(* Logix 5000 AddOnInstructionDefinition export POINT_DBL; software revision 30.00 *)

TYPE POINT :   // A point on an Edwards-curve represented in extended homogeneous coordinates
STRUCT
   X : DINT[22];
   Y : DINT[22];
   Z : DINT[22];
   T : DINT[22];
END_STRUCT
END_TYPE

ADD_ON_INSTRUCTION B256_ADD   (* revision 1.0 20170916, vendor Kenneth A. Fischer *)
// c3=c1+c2 with no reduction
// Revision note:
// Rev1.0: 20170916 - Initial Release
VAR_IN_OUT
   Inp_C1 : DINT[22]; {required}
   Inp_C2 : DINT[22]; {required}
   Out_C3 : DINT[22]; {required}
END_VAR
VAR
   i : INT;
END_VAR

ROUTINE Logic   (* ladder *)
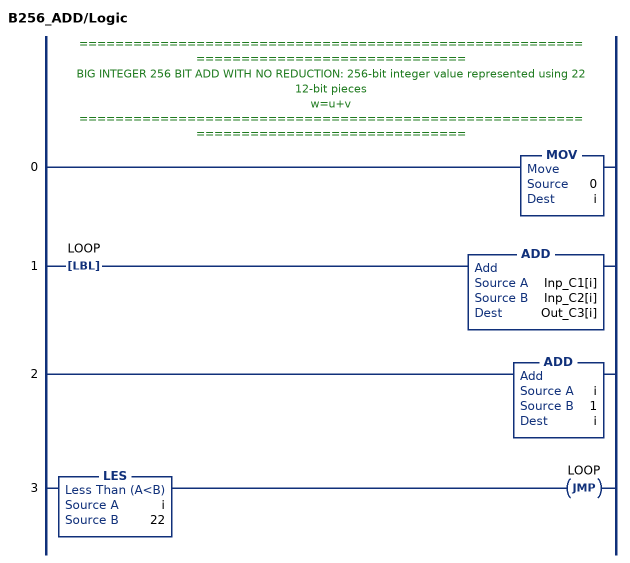
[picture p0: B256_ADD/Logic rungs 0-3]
   // ======================================================================================
   // BIG INTEGER 256 BIT ADD WITH NO REDUCTION: 256-bit integer value represented using 22 12-bit pieces
   // w=u+v
   // ======================================================================================
   0: MOV(0,i);
   1: LBL(LOOP)ADD(Inp_C1[i],Inp_C2[i],Out_C3[i]);
   2: ADD(i,1,i);
   3: LES(i,22)JMP(LOOP);
END_ROUTINE
END_ADD_ON_INSTRUCTION

ADD_ON_INSTRUCTION D_SHR   (* revision 1.0 20170524, vendor Kenneth A. Fischer *)
// DINT bit shift right of the 32-bit argument Inp_A by Inp_B bits with paddding by zeros on the right
// Revision note:
// Rev1.0: 20170524 - Initial Release
VAR_IN_OUT
   Inp_A : DINT; {required}   // 64-bit Integer to be right circular rotated
END_VAR
VAR_INPUT
   Inp_B : INT; {required}   // Number of bits to shift
END_VAR
VAR_IN_OUT
   Out : DINT; {required}   // Result
END_VAR
VAR
   BSR_Cntrl : CONTROL := (LEN := 32);
   ONS : BOOL;
   Source_Bit : BOOL;
   Wrk_InpA : DINT[2];
END_VAR

ROUTINE Logic   (* ladder *)
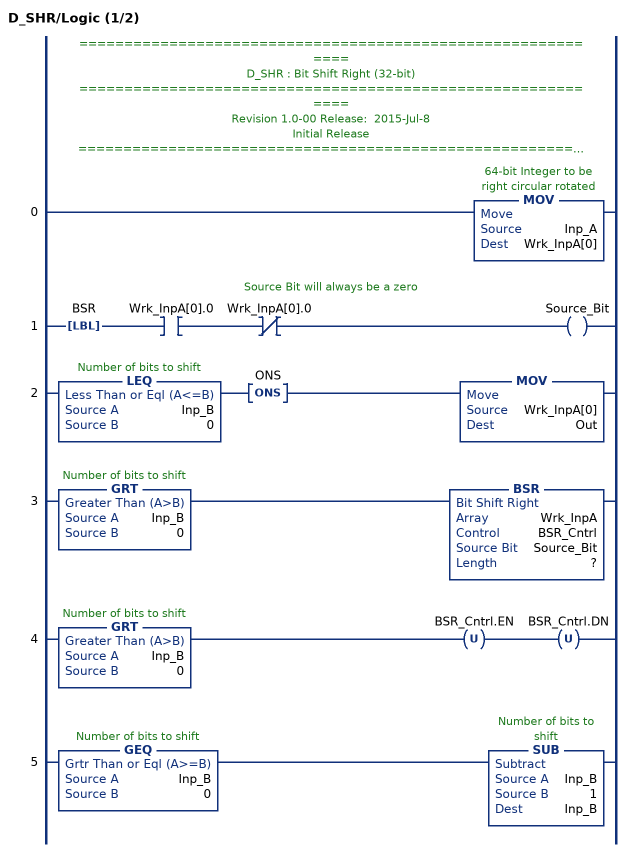
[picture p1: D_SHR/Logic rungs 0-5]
   // ============================================================
   // D_SHR : Bit Shift Right (32-bit)
   // ============================================================
   // Revision 1.0-00 Release:  2015-Jul-8
   // Initial Release
   // ============================================================
   // Performs a right bit shift of the 32-bit argument Inp_A by the
   // number of bits defined in the 16-bit argument Inp_B, with padding by zeros.
   0: MOV(Inp_A,Wrk_InpA[0]);
   // Source Bit will always be a zero
   1: LBL(BSR)XIC(Wrk_InpA[0].0)XIO(Wrk_InpA[0].0)OTE(Source_Bit);
   2: LEQ(Inp_B,0)ONS(ONS)MOV(Wrk_InpA[0],Out);
   3: GRT(Inp_B,0)BSR(Wrk_InpA,BSR_Cntrl,Source_Bit,?);
   4: GRT(Inp_B,0)OTU(BSR_Cntrl.EN)OTU(BSR_Cntrl.DN);
   5: GEQ(Inp_B,0)SUB(Inp_B,1,Inp_B);
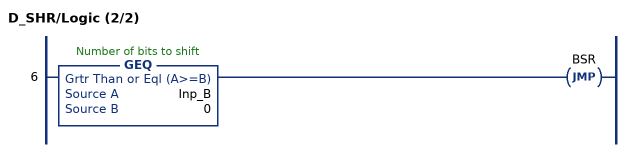
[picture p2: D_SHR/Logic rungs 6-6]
   6: GEQ(Inp_B,0)JMP(BSR);
END_ROUTINE
END_ADD_ON_INSTRUCTION

ADD_ON_INSTRUCTION B256_NRED   (* revision 1.0 20170916, vendor Kenneth A. Fischer *)
// Reduce 256-bit integer stored in 22 pieces by propagating carries
// Revision note:
// Rev1.0: 20170916 - Initial Release
VAR_IN_OUT
   Inp_C : DINT[22]; {required}
END_VAR
VAR
   D_SHR : D_SHR;
   temp : DINT;
   i : INT;
END_VAR

ROUTINE Logic   (* ladder *)
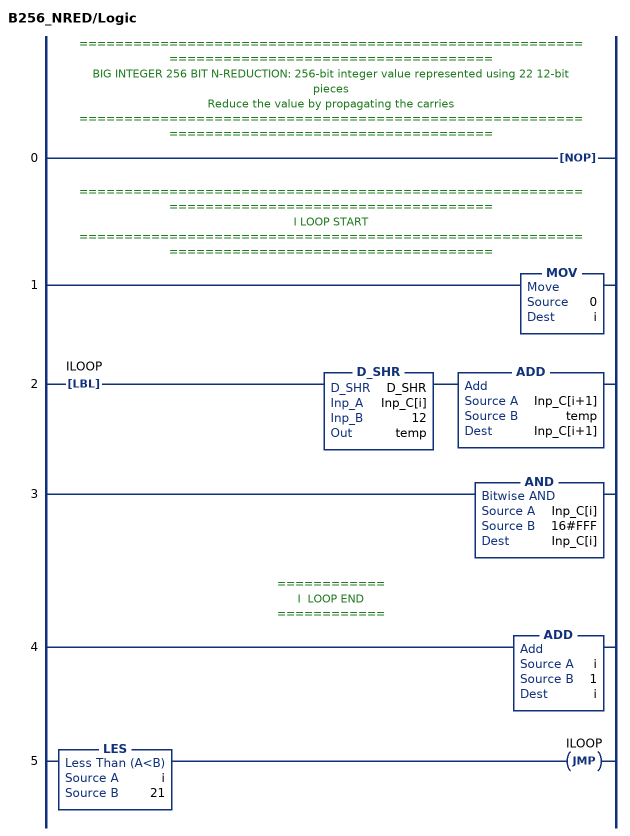
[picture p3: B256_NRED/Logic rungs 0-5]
   // ============================================================================================
   // BIG INTEGER 256 BIT N-REDUCTION: 256-bit integer value represented using 22 12-bit pieces
   // Reduce the value by propagating the carries
   // ============================================================================================
   0: NOP();
   // ============================================================================================
   // I LOOP START
   // ============================================================================================
   1: MOV(0,i);
   2: LBL(ILOOP)D_SHR(D_SHR,Inp_C[i],12,temp)ADD(Inp_C[i+1],temp,Inp_C[i+1]);
   3: AND(Inp_C[i],16#FFF,Inp_C[i]);
   // ============
   // I  LOOP END
   // ============
   4: ADD(i,1,i);
   5: LES(i,21)JMP(ILOOP);
END_ROUTINE
END_ADD_ON_INSTRUCTION

ADD_ON_INSTRUCTION B256_SUB   (* revision 1.0 20170916, vendor Kenneth A. Fischer *)
// c3=c1-c2 with reduction
// Revision note:
// Rev1.0: 20170916 - Initial Release
VAR_IN_OUT
   Inp_C1 : DINT[22]; {required}
   Inp_C2 : DINT[22]; {required}
   Out_C3 : DINT[22]; {required}
END_VAR
VAR
   B256_ADD : B256_ADD;
   B256_NRED : B256_NRED;
   temp : DINT;
   i : INT;
END_VAR

ROUTINE Logic   (* ladder *)
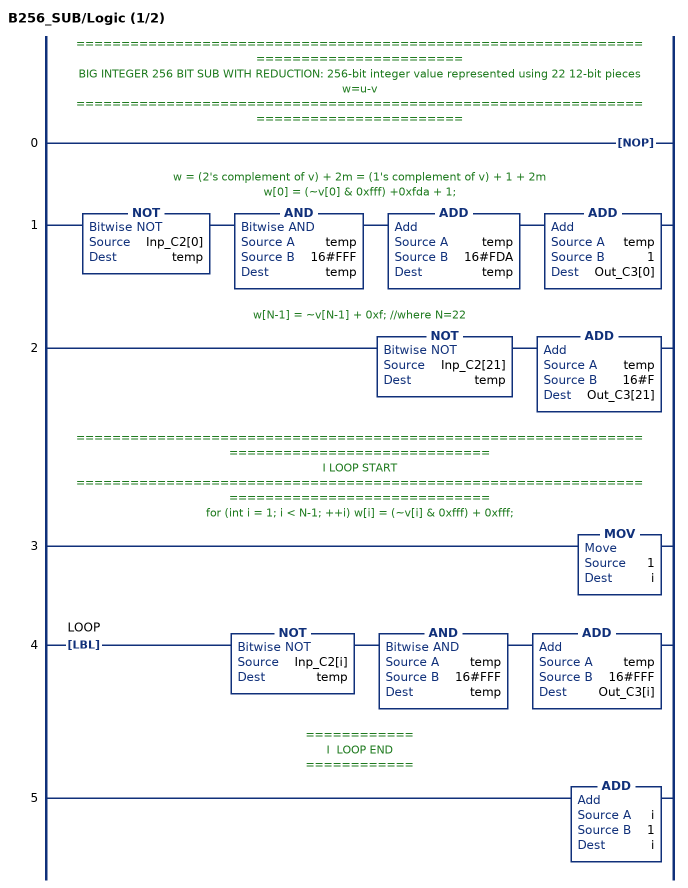
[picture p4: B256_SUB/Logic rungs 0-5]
   // ======================================================================================
   // BIG INTEGER 256 BIT SUB WITH REDUCTION: 256-bit integer value represented using 22 12-bit pieces
   //  w=u-v
   // ======================================================================================
   0: NOP();
   // w = (2's complement of v) + 2m = (1's complement of v) + 1 + 2m
   // w[0] = (~v[0] & 0xfff) +0xfda + 1;
   1: NOT(Inp_C2[0],temp)AND(temp,16#FFF,temp)ADD(temp,16#FDA,temp)ADD(temp,1,Out_C3[0]);
   // w[N-1] = ~v[N-1] + 0xf; //where N=22
   2: NOT(Inp_C2[21],temp)ADD(temp,16#F,Out_C3[21]);
   // ============================================================================================
   // I LOOP START
   // ============================================================================================
   // for (int i = 1; i < N-1; ++i) w[i] = (~v[i] & 0xfff) + 0xfff;
   3: MOV(1,i);
   4: LBL(LOOP)NOT(Inp_C2[i],temp)AND(temp,16#FFF,temp)ADD(temp,16#FFF,Out_C3[i]);
   // ============
   // I  LOOP END
   // ============
   5: ADD(i,1,i);
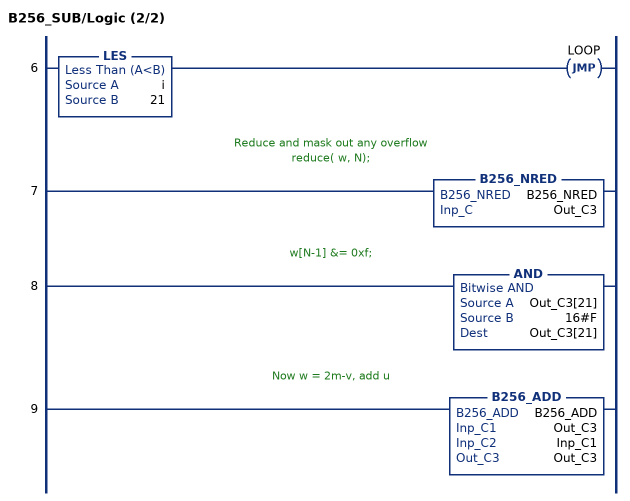
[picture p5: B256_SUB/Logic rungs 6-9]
   6: LES(i,21)JMP(LOOP);
   // Reduce and mask out any overflow
   // reduce( w, N);
   7: B256_NRED(B256_NRED,Out_C3);
   // w[N-1] &= 0xf;
   8: AND(Out_C3[21],16#F,Out_C3[21]);
   // Now w = 2m-v, add u
   9: B256_ADD(B256_ADD,Out_C3,Inp_C1,Out_C3);
END_ROUTINE
END_ADD_ON_INSTRUCTION

ADD_ON_INSTRUCTION B256_FRED   (* revision 1.0 20170916, vendor Kenneth A. Fischer *)
// fast_reduce:  reduce by propagating the carries starting at a particular offset and stoping once the carry becomes zero
// Revision note:
// Rev1.0: 20170916 - Initial Release
VAR_IN_OUT
   Inp_C : DINT[22]; {required}
END_VAR
VAR_INPUT
   Inp_offset : INT; {required}
END_VAR
VAR
   i : INT;
   carry : DINT;
   D_SHR : D_SHR;
END_VAR

ROUTINE Logic   (* ladder *)
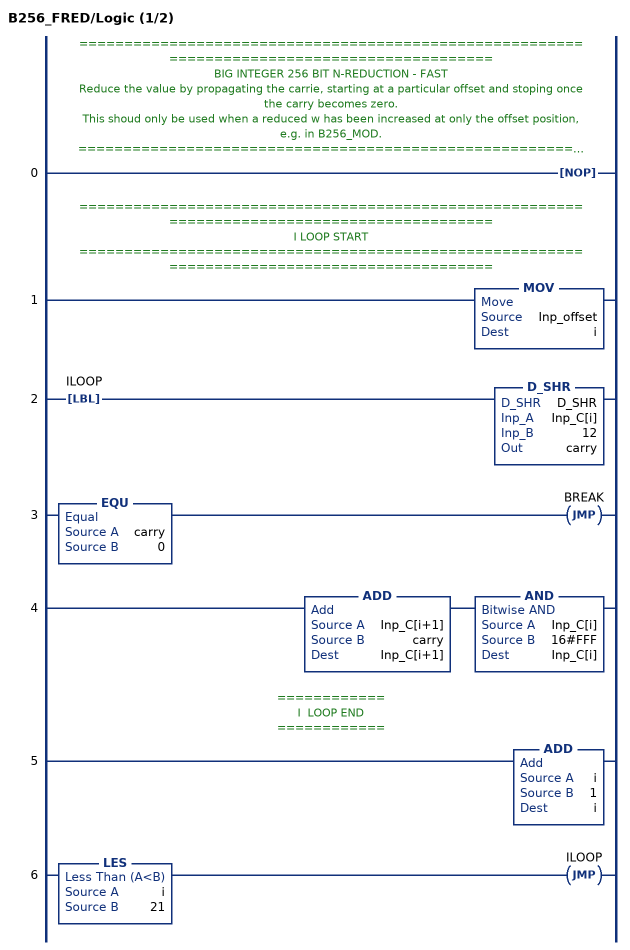
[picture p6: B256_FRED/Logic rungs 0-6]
   // ============================================================================================
   // BIG INTEGER 256 BIT N-REDUCTION - FAST
   // Reduce the value by propagating the carrie, starting at a particular offset and stoping once the carry becomes zero.
   // This shoud only be used when a reduced w has been increased at only the offset position, e.g. in B256_MOD.
   // ============================================================================================
   0: NOP();
   // ============================================================================================
   // I LOOP START
   // ============================================================================================
   1: MOV(Inp_offset,i);
   2: LBL(ILOOP)D_SHR(D_SHR,Inp_C[i],12,carry);
   3: EQU(carry,0)JMP(BREAK);
   4: ADD(Inp_C[i+1],carry,Inp_C[i+1])AND(Inp_C[i],16#FFF,Inp_C[i]);
   // ============
   // I  LOOP END
   // ============
   5: ADD(i,1,i);
   6: LES(i,21)JMP(ILOOP);
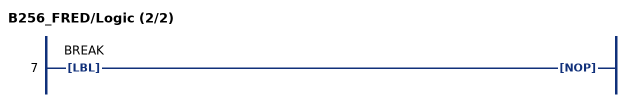
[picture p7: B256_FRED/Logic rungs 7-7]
   7: LBL(BREAK)NOP();
END_ROUTINE
END_ADD_ON_INSTRUCTION

ADD_ON_INSTRUCTION D_SHL   (* revision 1.0 20170524, vendor Kenneth A. Fischer *)
// DINT bit shift left of the 32-bit argument Inp_A by Inp_B bits with paddding by zeros on the right
// Revision note:
// Rev1.0: 20170524 - Initial Release
VAR_IN_OUT
   Inp_A : DINT; {required}   // 64-bit Integer to be right circular rotated
END_VAR
VAR_INPUT
   Inp_B : INT; {required}   // Number of bits to shift
END_VAR
VAR_IN_OUT
   Out : DINT; {required}   // Result
END_VAR
VAR
   Wrk_InpA : DINT[2];
   Source_Bit : BOOL;
   ONS : BOOL;
   BSL_Cntrl : CONTROL := (LEN := 32);
END_VAR

ROUTINE Logic   (* ladder *)
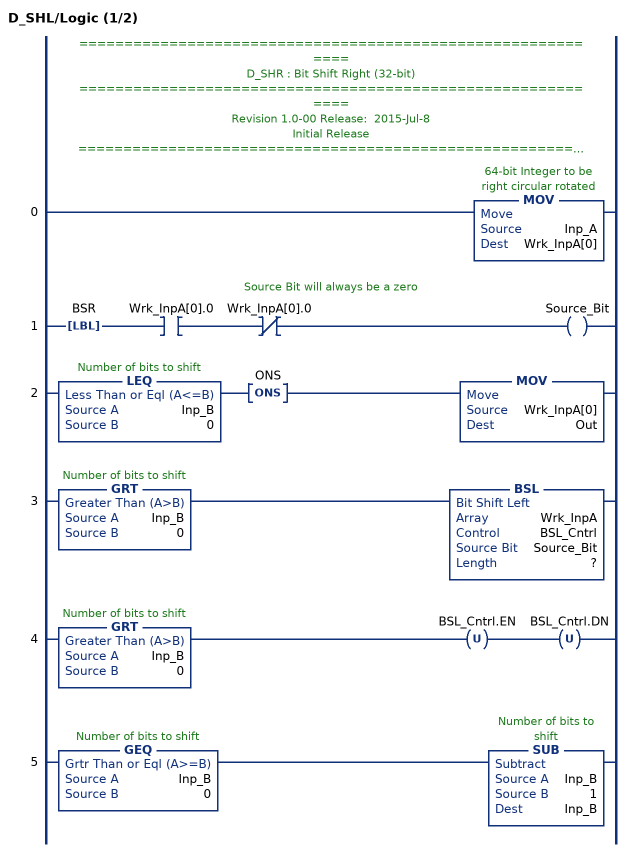
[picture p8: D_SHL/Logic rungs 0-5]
   // ============================================================
   // D_SHR : Bit Shift Right (32-bit)
   // ============================================================
   // Revision 1.0-00 Release:  2015-Jul-8
   // Initial Release
   // ============================================================
   // Performs a left bit shift of the 32-bit argument Inp_A by the
   // number of bits defined in the 16-bit argument Inp_B, with padding by zeros.
   0: MOV(Inp_A,Wrk_InpA[0]);
   // Source Bit will always be a zero
   1: LBL(BSR)XIC(Wrk_InpA[0].0)XIO(Wrk_InpA[0].0)OTE(Source_Bit);
   2: LEQ(Inp_B,0)ONS(ONS)MOV(Wrk_InpA[0],Out);
   3: GRT(Inp_B,0)BSL(Wrk_InpA,BSL_Cntrl,Source_Bit,?);
   4: GRT(Inp_B,0)OTU(BSL_Cntrl.EN)OTU(BSL_Cntrl.DN);
   5: GEQ(Inp_B,0)SUB(Inp_B,1,Inp_B);
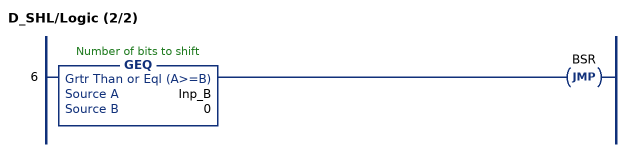
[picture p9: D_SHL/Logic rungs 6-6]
   6: GEQ(Inp_B,0)JMP(BSR);
END_ROUTINE
END_ADD_ON_INSTRUCTION

ADD_ON_INSTRUCTION B256_MOD   (* revision 1.0 20170916, vendor Kenneth A. Fischer *)
// c = d mod (2^255 - 19)
// Revision note:
// Rev1.0: 20170916 - Initial Release
VAR_IN_OUT
   Inp_D : DINT[43]; {required}
   Out_C : DINT[22]; {required}
END_VAR
VAR
   B256_NRED : B256_NRED;
   D_SHL : D_SHL;
   D_SHR : D_SHR;
   i : INT;
   t : DINT;
   temp : DINT;
   temp2 : DINT;
   B256_FRED : B256_FRED;
   offset : DINT;
END_VAR

ROUTINE Logic   (* ladder *)
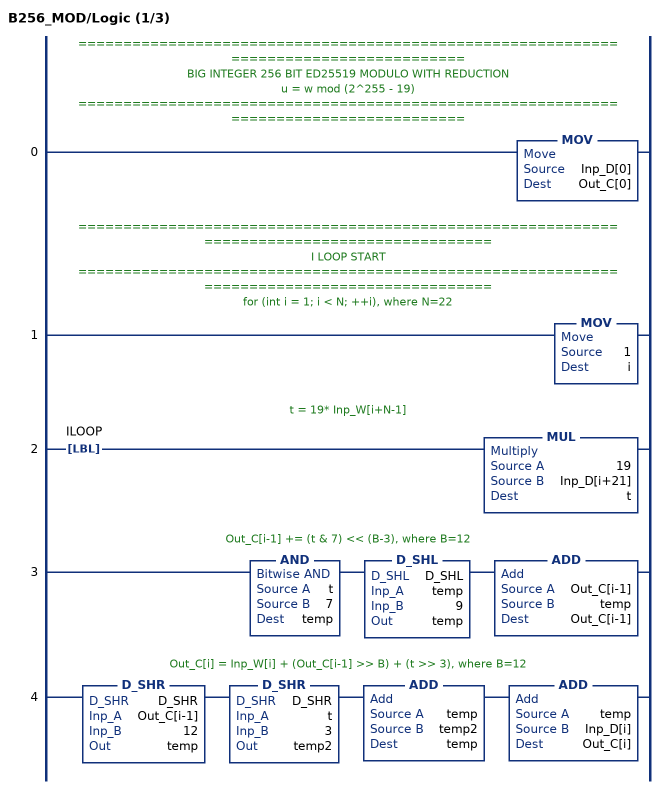
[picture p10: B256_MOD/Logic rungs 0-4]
   // ======================================================================================
   // BIG INTEGER 256 BIT ED25519 MODULO WITH REDUCTION
   //  u = w mod (2^255 - 19)
   // ======================================================================================
   0: MOV(Inp_D[0],Out_C[0]);
   // ============================================================================================
   // I LOOP START
   // ============================================================================================
   // for (int i = 1; i < N; ++i), where N=22
   1: MOV(1,i);
   // t = 19* Inp_W[i+N-1]
   2: LBL(ILOOP)MUL(19,Inp_D[i+21],t);
   // Out_C[i-1] += (t & 7) << (B-3), where B=12
   3: AND(t,7,temp)D_SHL(D_SHL,temp,9,temp)ADD(Out_C[i-1],temp,Out_C[i-1]);
   // Out_C[i] = Inp_W[i] + (Out_C[i-1] >> B) + (t >> 3), where B=12
   4: D_SHR(D_SHR,Out_C[i-1],12,temp)D_SHR(D_SHR,t,3,temp2)ADD(temp,temp2,temp)ADD(temp,Inp_D[i],Out_C[i]);
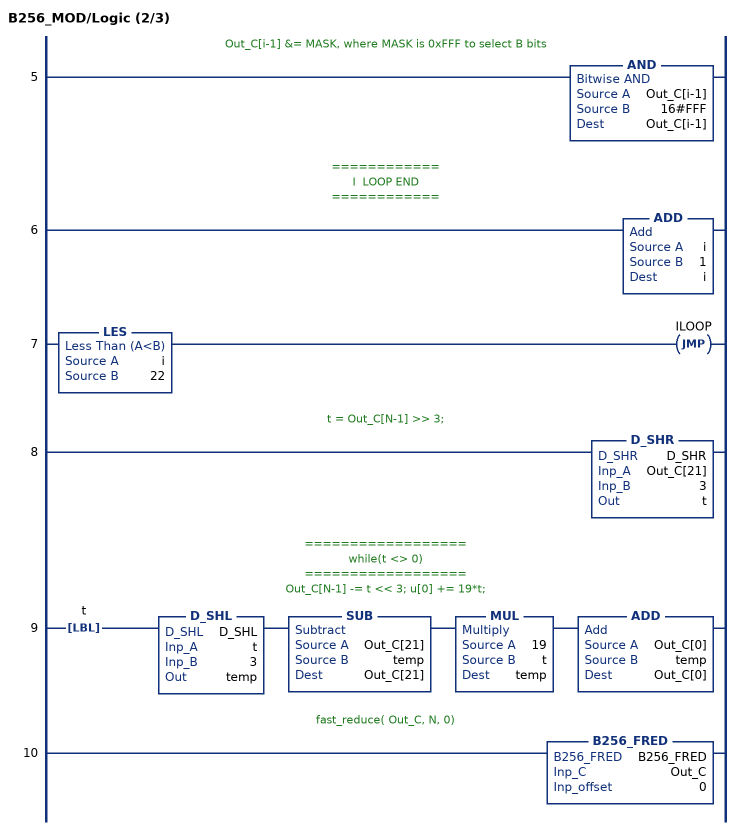
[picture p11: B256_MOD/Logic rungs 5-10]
   // Out_C[i-1] &= MASK, where MASK is 0xFFF to select B bits
   5: AND(Out_C[i-1],16#FFF,Out_C[i-1]);
   // ============
   // I  LOOP END
   // ============
   6: ADD(i,1,i);
   7: LES(i,22)JMP(ILOOP);
   // t = Out_C[N-1] >> 3;
   8: D_SHR(D_SHR,Out_C[21],3,t);
   // ==================
   // while(t <> 0)
   // ==================
   // Out_C[N-1] -= t << 3; u[0] += 19*t;
   9: LBL(t)D_SHL(D_SHL,t,3,temp)SUB(Out_C[21],temp,Out_C[21])MUL(19,t,temp)ADD(Out_C[0],temp,Out_C[0]);
   // fast_reduce( Out_C, N, 0)
   10: B256_FRED(B256_FRED,Out_C,0);
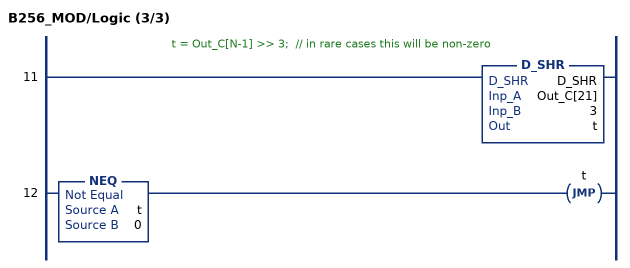
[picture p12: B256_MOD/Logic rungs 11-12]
   // t = Out_C[N-1] >> 3;  // in rare cases this will be non-zero
   11: D_SHR(D_SHR,Out_C[21],3,t);
   12: NEQ(t,0)JMP(t);
END_ROUTINE
END_ADD_ON_INSTRUCTION

ADD_ON_INSTRUCTION B256_NNRED   (* revision 1.0 20170916, vendor Kenneth A. Fischer *)
// Reduce 256-bit integer stored in 43 pieces by propagating carries
// Revision note:
// Rev1.0: 20170916 - Initial Release
VAR_IN_OUT
   Inp_D : DINT[43]; {required}
END_VAR
VAR
   temp : DINT;
   i : INT;
   D_SHR : D_SHR;
END_VAR

ROUTINE Logic   (* ladder *)
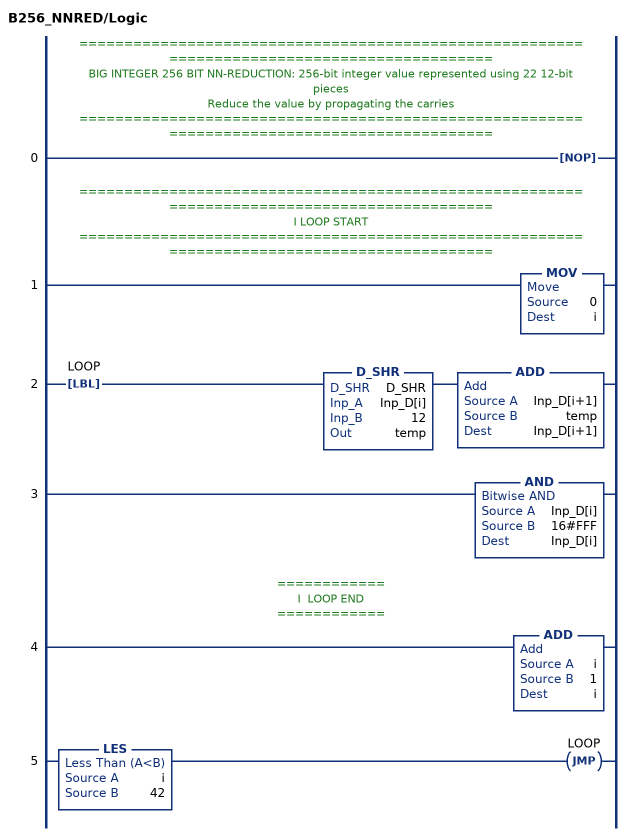
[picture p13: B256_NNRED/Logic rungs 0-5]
   // ============================================================================================
   // BIG INTEGER 256 BIT NN-REDUCTION: 256-bit integer value represented using 22 12-bit pieces
   // Reduce the value by propagating the carries
   // ============================================================================================
   0: NOP();
   // ============================================================================================
   // I LOOP START
   // ============================================================================================
   1: MOV(0,i);
   2: LBL(LOOP)D_SHR(D_SHR,Inp_D[i],12,temp)ADD(Inp_D[i+1],temp,Inp_D[i+1]);
   3: AND(Inp_D[i],16#FFF,Inp_D[i]);
   // ============
   // I  LOOP END
   // ============
   4: ADD(i,1,i);
   5: LES(i,42)JMP(LOOP);
END_ROUTINE
END_ADD_ON_INSTRUCTION

ADD_ON_INSTRUCTION B256_MUL   (* revision 1.0 20170916, vendor Kenneth A. Fischer *)
// c3 = c1*c2 with reduction and mod
// Revision note:
// Rev1.0: 20170916 - Initial Release
VAR_IN_OUT
   Temp_D : DINT[43]; {required}
   Inp_C1 : DINT[22]; {required}
   Inp_C2 : DINT[22]; {required}
   Out_C3 : DINT[22]; {required}
END_VAR
VAR
   B256_MOD : B256_MOD;
   B256_NNRED : B256_NNRED;
   i : INT;
   j : INT;
   mul_temp : DINT;
END_VAR

ROUTINE Logic   (* ladder *)
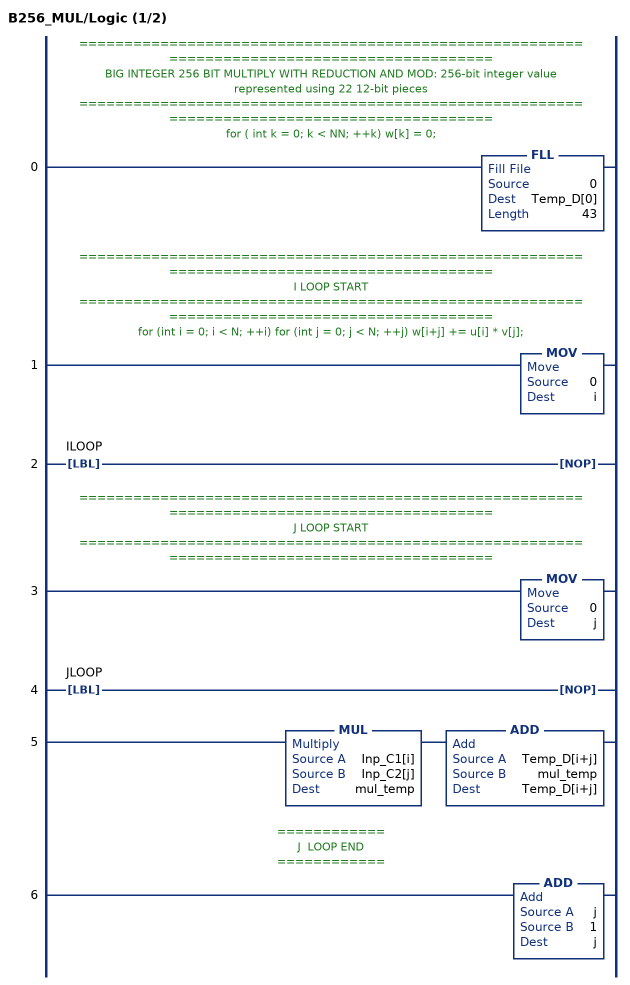
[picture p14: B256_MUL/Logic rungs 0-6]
   // ============================================================================================
   // BIG INTEGER 256 BIT MULTIPLY WITH REDUCTION AND MOD: 256-bit integer value represented using 22 12-bit pieces
   // ============================================================================================
   // for ( int k = 0; k < NN; ++k) w[k] = 0;
   0: FLL(0,Temp_D[0],43);
   // ============================================================================================
   // I LOOP START
   // ============================================================================================
   // for (int i = 0; i < N; ++i) for (int j = 0; j < N; ++j) w[i+j] += u[i] * v[j];
   1: MOV(0,i);
   2: LBL(ILOOP)NOP();
   // ============================================================================================
   // J LOOP START
   // ============================================================================================
   3: MOV(0,j);
   4: LBL(JLOOP)NOP();
   5: MUL(Inp_C1[i],Inp_C2[j],mul_temp)ADD(Temp_D[i+j],mul_temp,Temp_D[i+j]);
   // ============
   // J  LOOP END
   // ============
   6: ADD(j,1,j);
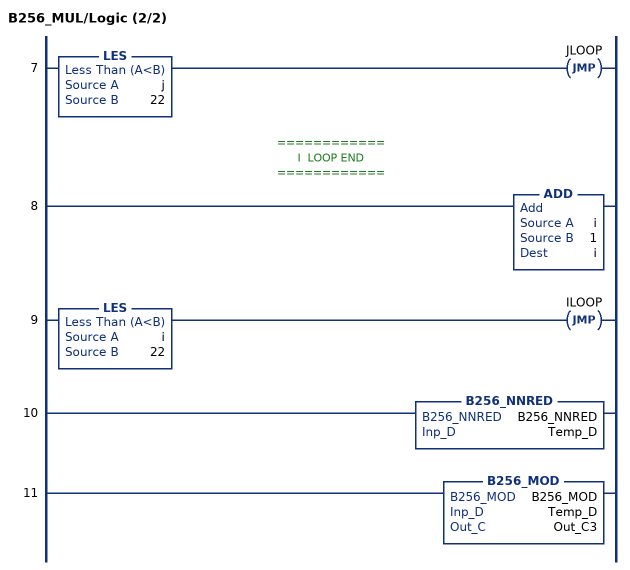
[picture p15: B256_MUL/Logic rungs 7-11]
   7: LES(j,22)JMP(JLOOP);
   // ============
   // I  LOOP END
   // ============
   8: ADD(i,1,i);
   9: LES(i,22)JMP(ILOOP);
   10: B256_NNRED(B256_NNRED,Temp_D);
   11: B256_MOD(B256_MOD,Temp_D,Out_C3);
END_ROUTINE
END_ADD_ON_INSTRUCTION

ADD_ON_INSTRUCTION B256_MUL2   (* revision 1.0 20170916, vendor Kenneth A. Fischer *)
// c3= 2*c1*c2 with reduction and mod
// Revision note:
// Rev1.0: 20170916 - Initial Release
VAR_IN_OUT
   Temp_D : DINT[43]; {required}
   Inp_C1 : DINT[22]; {required}
   Inp_C2 : DINT[22]; {required}
   Out_C3 : DINT[22]; {required}
END_VAR
VAR
   B256_NNRED : B256_NNRED;
   i : INT;
   j : INT;
   mul_temp : DINT;
   B256_MOD : B256_MOD;
   t : DINT;
END_VAR

ROUTINE Logic   (* ladder *)
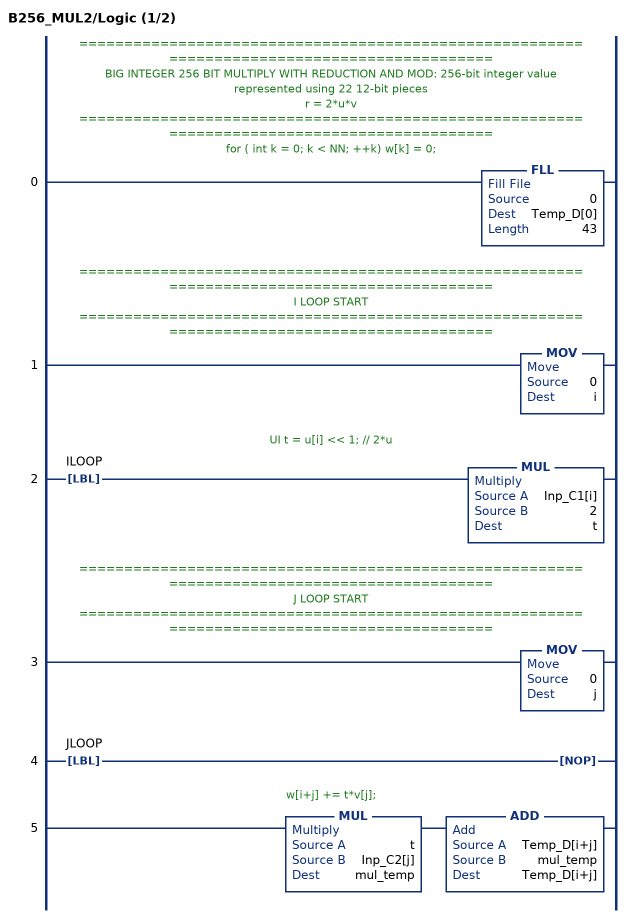
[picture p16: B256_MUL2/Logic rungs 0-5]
   // ============================================================================================
   // BIG INTEGER 256 BIT MULTIPLY WITH REDUCTION AND MOD: 256-bit integer value represented using 22 12-bit pieces
   // r = 2*u*v
   // ============================================================================================
   // for ( int k = 0; k < NN; ++k) w[k] = 0;
   0: FLL(0,Temp_D[0],43);
   // ============================================================================================
   // I LOOP START
   // ============================================================================================
   1: MOV(0,i);
   // UI t = u[i] << 1; // 2*u
   2: LBL(ILOOP)MUL(Inp_C1[i],2,t);
   // ============================================================================================
   // J LOOP START
   // ============================================================================================
   3: MOV(0,j);
   4: LBL(JLOOP)NOP();
   // w[i+j] += t*v[j];
   5: MUL(t,Inp_C2[j],mul_temp)ADD(Temp_D[i+j],mul_temp,Temp_D[i+j]);
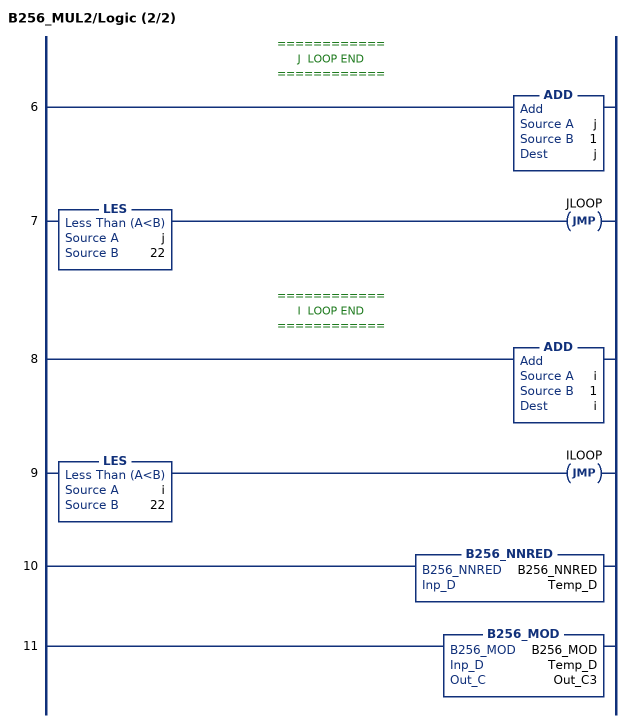
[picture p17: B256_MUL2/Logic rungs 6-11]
   // ============
   // J  LOOP END
   // ============
   6: ADD(j,1,j);
   7: LES(j,22)JMP(JLOOP);
   // ============
   // I  LOOP END
   // ============
   8: ADD(i,1,i);
   9: LES(i,22)JMP(ILOOP);
   10: B256_NNRED(B256_NNRED,Temp_D);
   11: B256_MOD(B256_MOD,Temp_D,Out_C3);
END_ROUTINE
END_ADD_ON_INSTRUCTION

ADD_ON_INSTRUCTION B256_SQU   (* revision 1.0 20170916, vendor Kenneth A. Fischer *)
// c2 = c1*c1 with reduction and mod
// uses about half the number of multiplies compared to B256_MOD
// Revision note:
// Rev1.0: 20170916 - Initial Release
VAR_IN_OUT
   Temp_D : DINT[43]; {required}
   Inp_C1 : DINT[22]; {required}
   Out_C2 : DINT[22]; {required}
END_VAR
VAR
   B256_NNRED : B256_NNRED;
   i : INT;
   j : INT;
   z : INT;
   mul_temp : DINT;
   B256_MOD : B256_MOD;
   B256_NRED : B256_NRED;
   t : DINT;
END_VAR

ROUTINE Logic   (* ladder *)
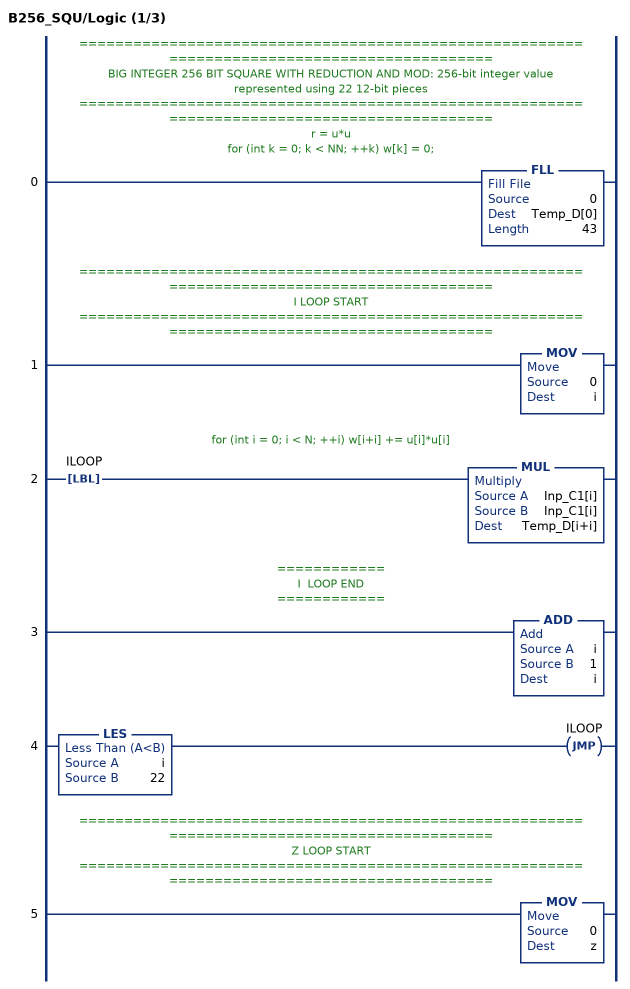
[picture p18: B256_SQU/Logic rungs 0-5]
   // ============================================================================================
   // BIG INTEGER 256 BIT SQUARE WITH REDUCTION AND MOD: 256-bit integer value represented using 22 12-bit pieces
   // ============================================================================================
   // r = u*u
   // for (int k = 0; k < NN; ++k) w[k] = 0;
   0: FLL(0,Temp_D[0],43);
   // ============================================================================================
   // I LOOP START
   // ============================================================================================
   1: MOV(0,i);
   // for (int i = 0; i < N; ++i) w[i+i] += u[i]*u[i]
   2: LBL(ILOOP)MUL(Inp_C1[i],Inp_C1[i],Temp_D[i+i]);
   // ============
   // I  LOOP END
   // ============
   3: ADD(i,1,i);
   4: LES(i,22)JMP(ILOOP);
   // ============================================================================================
   // Z LOOP START
   // ============================================================================================
   5: MOV(0,z);
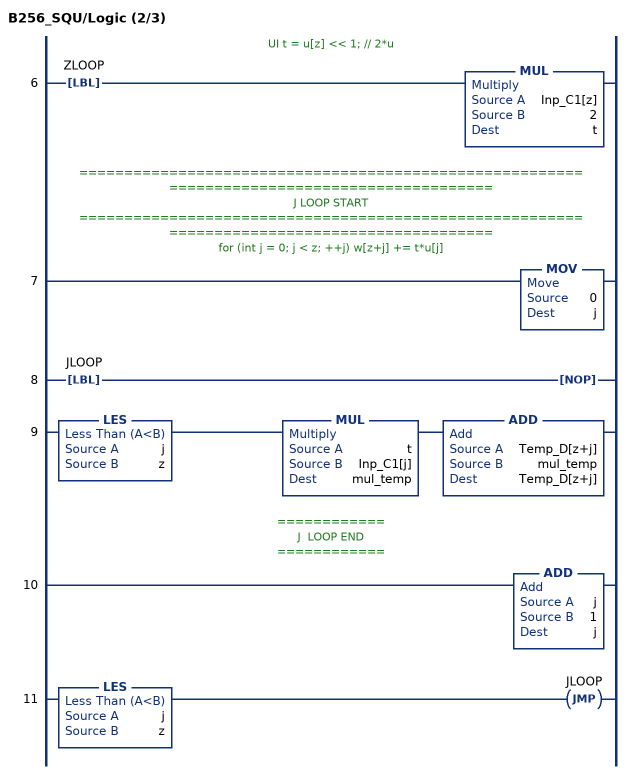
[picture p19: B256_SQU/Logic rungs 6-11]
   // UI t = u[z] << 1; // 2*u
   6: LBL(ZLOOP)MUL(Inp_C1[z],2,t);
   // ============================================================================================
   // J LOOP START
   // ============================================================================================
   // for (int j = 0; j < z; ++j) w[z+j] += t*u[j]
   7: MOV(0,j);
   8: LBL(JLOOP)NOP();
   9: LES(j,z)MUL(t,Inp_C1[j],mul_temp)ADD(Temp_D[z+j],mul_temp,Temp_D[z+j]);
   // ============
   // J  LOOP END
   // ============
   10: ADD(j,1,j);
   11: LES(j,z)JMP(JLOOP);
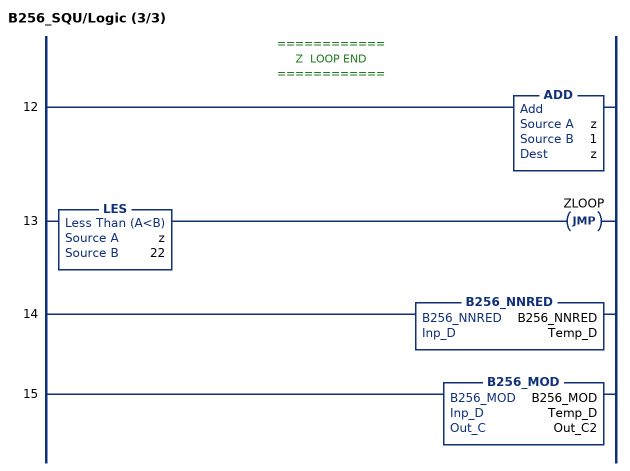
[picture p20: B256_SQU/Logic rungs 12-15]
   // ============
   // Z  LOOP END
   // ============
   12: ADD(z,1,z);
   13: LES(z,22)JMP(ZLOOP);
   14: B256_NNRED(B256_NNRED,Temp_D);
   15: B256_MOD(B256_MOD,Temp_D,Out_C2);
END_ROUTINE
END_ADD_ON_INSTRUCTION

ADD_ON_INSTRUCTION POINT_DBL   (* revision 1.0 20170916, vendor Kenneth A. Fischer *)
// Point Doubling:
// p3 = p1 + p1
// Requires POINT UDT
// Revision note:
// Rev1.0: 20170916 - Initial Release
VAR_IN_OUT
   Temp_C1 : DINT[22]; {required}   // A
   Temp_C2 : DINT[22]; {required}   // B
   Temp_C3 : DINT[22]; {required}   // C
   Temp_C4 : DINT[22]; {required}   // D
   Temp_C5 : DINT[22]; {required}   // F
   Temp_C6 : DINT[22]; {required}   // G
   Temp_C7 : DINT[22]; {required}   // H
   Temp_C8 : DINT[22]; {required}   // R
   Temp_C9 : DINT[22]; {required}   // S
   Temp_D : DINT[43]; {required}   // W
   Inp_P1 : POINT; {required}
   Out_P3 : POINT; {required}
END_VAR
VAR
   B256_ADD : B256_ADD;
   B256_MUL : B256_MUL;
   B256_SUB : B256_SUB;
   B256_MUL2 : B256_MUL2;
   B256_SQR : B256_SQU;
END_VAR

ROUTINE Logic   (* ladder *)
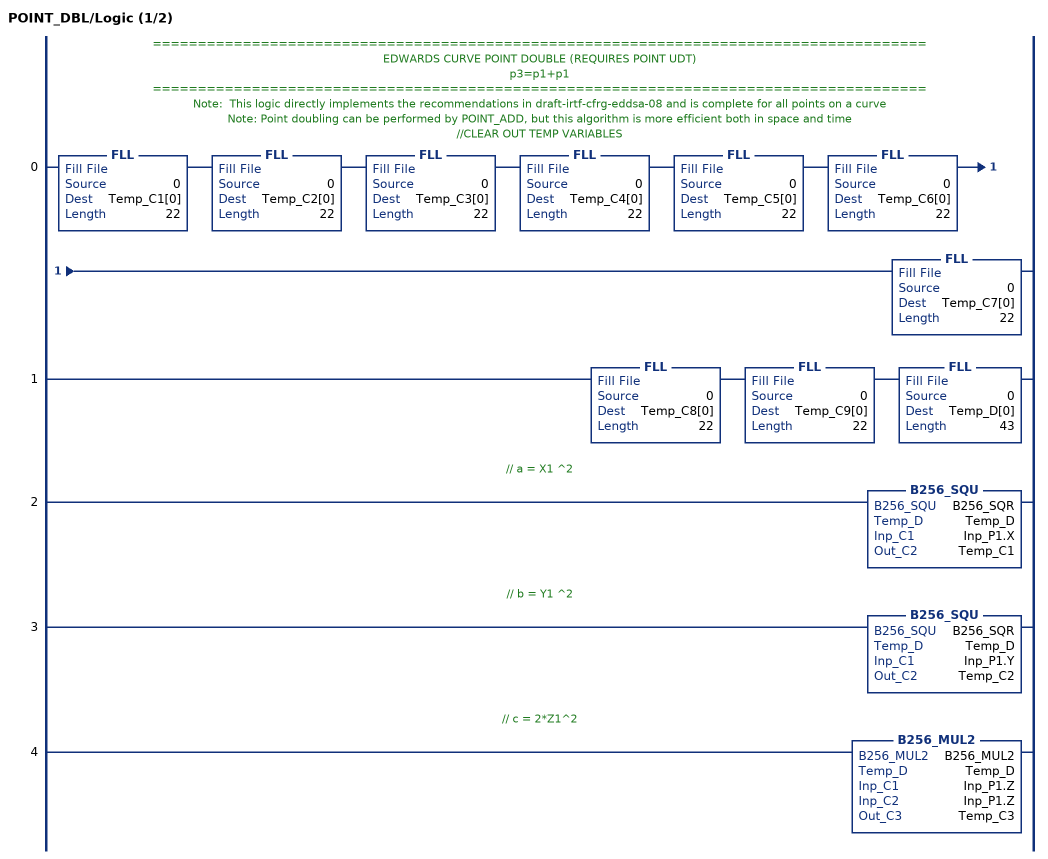
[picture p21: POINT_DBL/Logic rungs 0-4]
   // ======================================================================================
   // EDWARDS CURVE POINT DOUBLE (REQUIRES POINT UDT)
   // p3=p1+p1
   // ======================================================================================
   // Note:  This logic directly implements the recommendations in draft-irtf-cfrg-eddsa-08 and is complete for all points on a curve
   // Note: Point doubling can be performed by POINT_ADD, but this algorithm is more efficient both in space and time
   // //CLEAR OUT TEMP VARIABLES
   0: FLL(0,Temp_C1[0],22)FLL(0,Temp_C2[0],22)FLL(0,Temp_C3[0],22)FLL(0,Temp_C4[0],22)FLL(0,Temp_C5[0],22)FLL(0,Temp_C6[0],22)FLL(0,Temp_C7[0],22);
   1: FLL(0,Temp_C8[0],22)FLL(0,Temp_C9[0],22)FLL(0,Temp_D[0],43);
   // // a = X1 ^2
   2: B256_SQU(B256_SQR,Temp_D,Inp_P1.X,Temp_C1);
   // // b = Y1 ^2
   3: B256_SQU(B256_SQR,Temp_D,Inp_P1.Y,Temp_C2);
   // // c = 2*Z1^2
   4: B256_MUL2(B256_MUL2,Temp_D,Inp_P1.Z,Inp_P1.Z,Temp_C3);
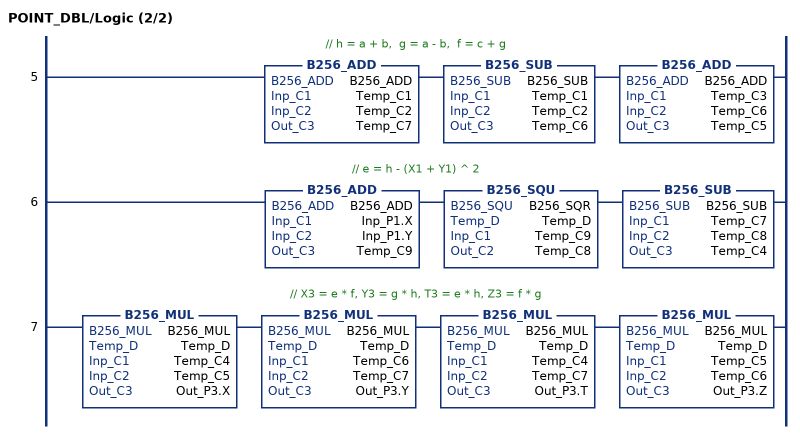
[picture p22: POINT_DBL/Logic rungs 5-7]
   // // h = a + b,  g = a - b,  f = c + g
   5: B256_ADD(B256_ADD,Temp_C1,Temp_C2,Temp_C7)B256_SUB(B256_SUB,Temp_C1,Temp_C2,Temp_C6)B256_ADD(B256_ADD,Temp_C3,Temp_C6,Temp_C5);
   // // e = h - (X1 + Y1) ^ 2
   6: B256_ADD(B256_ADD,Inp_P1.X,Inp_P1.Y,Temp_C9)B256_SQU(B256_SQR,Temp_D,Temp_C9,Temp_C8)B256_SUB(B256_SUB,Temp_C7,Temp_C8,Temp_C4);
   // // X3 = e * f, Y3 = g * h, T3 = e * h, Z3 = f * g
   7: B256_MUL(B256_MUL,Temp_D,Temp_C4,Temp_C5,Out_P3.X)B256_MUL(B256_MUL,Temp_D,Temp_C6,Temp_C7,Out_P3.Y)B256_MUL(B256_MUL,Temp_D,Temp_C4,Temp_C7,Out_P3.T)B256_MUL(B256_MUL,Temp_D,Temp_C5,Temp_C6,Out_P3.Z);
END_ROUTINE
END_ADD_ON_INSTRUCTION
